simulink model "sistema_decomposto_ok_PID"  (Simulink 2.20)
settings: Solver=ode45  StartTime=0.0  StopTime=10.0  RelTol=1e-3  AbsTol=1e-6
libraries: simulink_extras x1

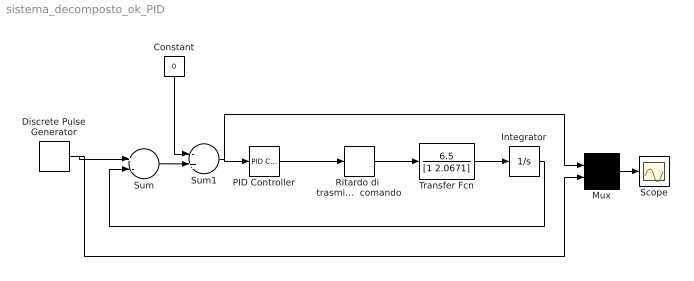
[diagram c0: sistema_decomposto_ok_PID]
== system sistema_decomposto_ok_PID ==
  Constant : Constant  Orientation=down  Value=0
  Discrete Pulse Generator : DiscretePulseGenerator  Amplitude=47.5  Period=100  PulseWidth=100  PhaseDelay=10  SampleTime=.1
  Integrator : Integrator  ExternalReset=none  InitialConditionSource=internal  InitialCondition=0  LimitOutput=off  UpperSaturationLimit=inf  LowerSaturationLimit=-inf  ShowSaturationPort=off  ShowStatePort=off  AbsoluteTolerance=auto
  Mux : Mux  Inputs=2
  PID Controller : simulink_extras/Additional Linear/PID Controller  P=0.9  I=0  D=0.35
  Ritardo di  trasmissione  comando : TransportDelay  DelayTime=.190  InitialInput=0  BufferSize=1024
  Scope : Scope
  Sum : Sum  Inputs=+-
  Sum1 : Sum  Inputs=-+
  Transfer Fcn : TransferFcn  Numerator=6.5  Denominator=[1 2.0671]
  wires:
  Discrete Pulse Generator/1 -> Sum/1, Mux/2
  Sum/1 -> Sum1/2
  Constant/1 -> Sum1/1
  Sum1/1 -> Mux/1, PID Controller/1
  Mux/1 -> Scope/1
  Transfer Fcn/1 -> Integrator/1
  Integrator/1 -> Sum/2
  PID Controller/1 -> Ritardo di  trasmissione  comando/1
  Ritardo di  trasmissione  comando/1 -> Transfer Fcn/1
